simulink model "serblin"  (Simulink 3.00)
settings: Solver=ode45  StartTime=0.0  StopTime=20  MaxStep=0.01  RelTol=1e-5  AbsTol=1e-5
undefined symbols (not defined in the file or in its folder): alfa, hbar, hiniz, S, ubar

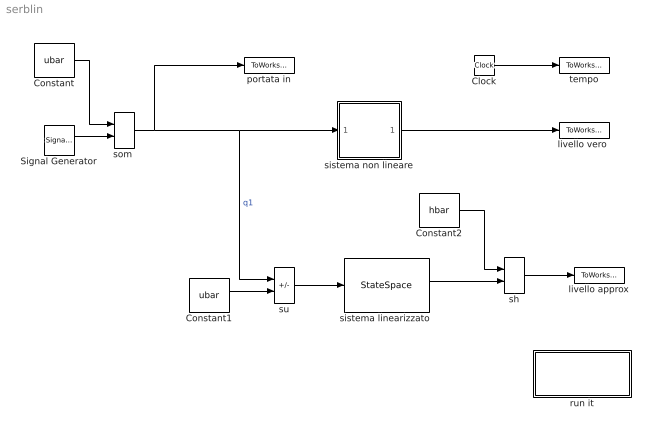
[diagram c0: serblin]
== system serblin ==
  Clock : Clock
  Constant : Constant  Value=ubar
  Constant1 : Constant  Value=ubar
  Constant2 : Constant  Value=hbar
  Signal Generator : SignalGenerator  WaveForm=sine  Amplitude=0.5  Frequency=0.2  Units=Hertz
  livello approx : ToWorkspace  VariableName=hlin  SampleTime=0  SaveFormat=Matrix
  "livello vero " : ToWorkspace  VariableName=h  SampleTime=0  SaveFormat=Matrix
  portata in : ToWorkspace  VariableName=q1  SampleTime=0  SaveFormat=Matrix
  run it : Subsystem  Description=confronto
  sh : Sum  Inputs=++  SaturateOnIntegerOverflow=on
  "sistema linearizzato " : StateSpace  A=-(alfa^2)/(2*S*ubar)  B=1/S  C=1  D=0  X0=hiniz-hbar
  sistema non lineare : Subsystem
  "som " : Sum  Inputs=++  SaturateOnIntegerOverflow=on
  su : Sum  Inputs=+-  SaturateOnIntegerOverflow=on
  tempo : ToWorkspace  VariableName=t  SampleTime=0  SaveFormat=Matrix
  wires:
  Constant/1 -> "som "/1
  Signal Generator/1 -> "som "/2
  "som "/1 -> portata in/1, sistema non lineare/1(In1), su/1  "q1"
  sistema non lineare/1(Out1) -> "livello vero "/1
  Clock/1 -> tempo/1
  su/1 -> "sistema linearizzato "/1
  Constant1/1 -> su/2
  sh/1 -> livello approx/1
  "sistema linearizzato "/1 -> sh/2
  Constant2/1 -> sh/1

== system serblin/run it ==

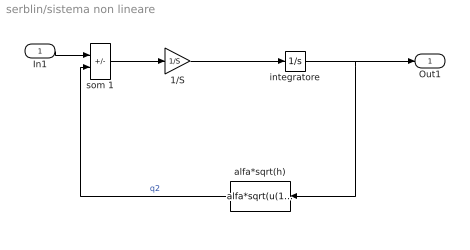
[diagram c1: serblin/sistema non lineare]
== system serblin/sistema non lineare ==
  In1 : Inport  Port=1  PortWidth=-1  SampleTime=-1  DataType=auto
  1/S : Gain  Gain=1/S  SaturateOnIntegerOverflow=on
  alfa*sqrt(h) : Fcn  Orientation=left  Expr=alfa*sqrt(u(1))
  integratore : Integrator  ExternalReset=none  InitialConditionSource=internal  InitialCondition=hiniz  LimitOutput=off  UpperSaturationLimit=inf  LowerSaturationLimit=-inf  ShowSaturationPort=off  ShowStatePort=off  AbsoluteTolerance=auto
  som 1 : Sum  Inputs=+-  SaturateOnIntegerOverflow=on
  Out1 : Outport  Port=1
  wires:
  som 1/1 -> 1/S/1
  In1/1 -> som 1/1
  1/S/1 -> integratore/1
  integratore/1 -> alfa*sqrt(h)/1, Out1/1
  alfa*sqrt(h)/1 -> som 1/2  "q2"
